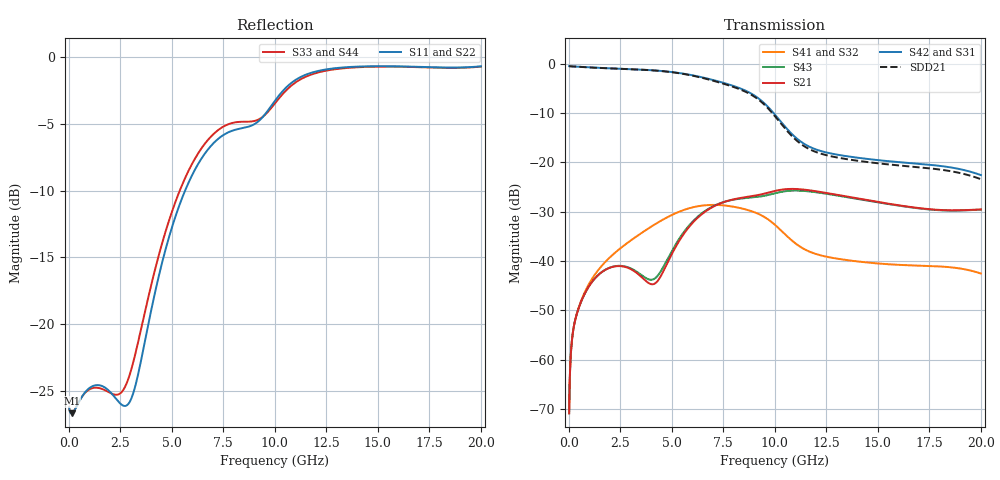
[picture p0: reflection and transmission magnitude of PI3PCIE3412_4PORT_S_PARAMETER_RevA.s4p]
! NPort=4 DATA=800 NOISE=0 GROUPDELAY=0 COMPLEX_DATAFORMAT=POLAR
! NumOfBlock=1 NumOfParam=0
! .MODEL Smodel S TSTONEFILE=PI3PCIE3412_4PORT_S_PARAMETER_RevA.s4p TYPE=S
!  -- The above .MODEL line can be used for the S element in the netlist.
! PORT DEFINITION
! PORT1 = INPUT+
! PORT2 = INPUT-
! PORT3 = OUTPUT+
! PORT4 = OUTPUT-
# Hz S MA R  50
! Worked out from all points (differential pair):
!   800 points, 25 MHz to 20 GHz, reference 50 ohm
!   strongest paths, dB at 25 MHz, 5.025 GHz, 10.03 GHz, 15.03 GHz, 20 GHz:
!     S42: -0.5, -1.7, -10.4, -19.5, -22.6
!     S31: -0.5, -1.7, -10.4, -19.6, -22.6
!     S21: -70.9, -38.5, -25.8, -28.0, -29.5
!     S43: -70.9, -37.9, -26.2, -28.1, -29.6
!     S41: -70.9, -30.6, -32.7, -40.5, -42.5
!     S32: -70.9, -30.6, -32.7, -40.5, -42.5
!   taken as a pair (ports 2,1 in; 4,3 out), SDD21 dB: -0.5, -1.7, -10.7, -20.2, -23.4
!   lowest |S11| = -26.7 dB at 150 MHz (marker M1), VSWR 1.10, Z = 54.8 - j0.43 ohm
!   |S11| at or under -10 dB: start of sweep to 5.652 GHz
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2.5e7  0.04861 -3.1  0.0002854 85.9  0.9477 -0.7  0.0002847 85.9
       0.0002854 85.9  0.04864 -3.1  0.0002847 85.9  0.9477 -0.7
       0.9477 -0.7  0.0002847 85.9  0.04864 -2.9  0.0002854 85.9
       0.0002847 85.9  0.9477 -0.7  0.0002854 85.9  0.04862 -2.9
1.5e8  0.04624 -4.9  0.001487 70.9  0.9433 -3.5  0.001485 70.7
       0.001487 70.9  0.04628 -4.8  0.001485 70.7  0.9433 -3.5
       0.9433 -3.5  0.001485 70.7  0.0463 -3.5  0.001487 70.9
       0.001485 70.7  0.9433 -3.5  0.001487 71.0  0.04626 -3.5
1.5e9  0.05889 -49.1  0.007401 51.5  0.9106 -31.2  0.008398 48.7
       0.007399 51.4  0.05888 -48.7  0.008401 48.8  0.9106 -31.2
       0.9105 -31.2  0.008401 48.8  0.05747 -38.5  0.007404 52.2
       0.008398 48.7  0.9107 -31.2  0.007407 52.2  0.05744 -38.9
3.85e9  0.09823 -13.5  0.006041 49.2  0.8665 -79.5  0.02125 6.8
        0.00603 49.3  0.09909 -13.5  0.02127 6.8  0.8664 -79.5
        0.8663 -79.5  0.02127 6.8  0.1243 -10.9  0.006532 52.7
        0.02125 6.8  0.8666 -79.5  0.006543 52.6  0.1235 -11.0
7.075e9  0.48 -56.9  0.03606 68.9  0.6802 -154.3  0.03707 -83.2
         0.03609 68.9  0.4809 -57.0  0.03708 -83.3  0.6802 -154.3
         0.6799 -154.3  0.03709 -83.3  0.5191 -59.1  0.03648 65.4
         0.03707 -83.2  0.6805 -154.3  0.03646 65.4  0.5181 -59.1
9.5e9  0.607 -75.2  0.04826 33.7  0.3968 140.4  0.02794 -156.6
       0.04825 33.7  0.6067 -75.2  0.02793 -156.6  0.3971 140.3
       0.3966 140.3  0.02793 -156.6  0.6052 -79.5  0.04585 31.2
       0.02794 -156.6  0.3973 140.4  0.04586 31.2  0.6042 -79.5
2e10  0.9241 -133.1  0.03334 -31.2  0.07433 44.7  0.007459 69.2
      0.03334 -31.2  0.9239 -133.1  0.00746 69.2  0.07432 44.3
      0.07424 44.5  0.007459 69.2  0.9216 -133.2  0.03319 -30.9
      0.00746 69.2  0.07441 44.5  0.03319 -30.9  0.9217 -133.2
